|   This file is an IBIS representation of the   |
|   Integrated Device Technology Inc   |
|   IDT8T49N1012   |
|   FEMTOCLOCK NG 12-OUTPUT UNIVERSAL FREQUENCY SYNTHESIZER   |
[IBIS Ver]   4.1
[File name]   8t49n1012.ibs
[File Rev]   1.0
[Date]   16 Oct 2015
[Source]   Originated at Integrated Device Technology, Inc.
[Disclaimer]
IDT hereby grants the user of this IBIS model a non-exclusive,
nontransferable license to use this IBIS model under the following terms.
Before using this IBIS model, the user should read this license.
If the user does not accept these terms,  the IBIS model should be
returned to IDT within 30 days.
   The user is granted this license only to use the IBIS model and
is not granted rights to sell, load, rent, lease or license the IBIS
model in whole or in part, or in modified form to anyone other than
user. User may modify the IBIS model to suit its specific
applications but rights to derivative works and such modifications
shall belong to IDT.
   This IBIS model is provided on an "AS IS" basis and IDT makes
absolutely no warranty with respect to the information contained
herein. IDT DISCLAIMS AND CUSTOMER WAIVES ALL WARRANTIES, EXPRESS
OR IMPLIED, INCLUDING WARRANTIES OF MERCHANTABILITY OR FITNESS FOR
A PARTICULAR PURPOSE. The entire risk as to quality and performance
is with the Customer. ACCORDINGLY, IN NO EVENT SHALL THE COMPANY BE
LIABLE FOR ANY DAMAGES, WHETHER IN CONTRACT OR TORT,INCLUDING ANY
LOST PROFITS OR OTHER INCIDENTAL, CONSEQUENTIAL, EXEMPLARY, OR
PUNITIVE DAMAGES ARISING OUT OF THE USE OR APPLICATION OF THE IBIS
model provided in this package. Further, IDT reserves the right to
make changes without notice to any product herein to improve
reliability, function, or design. IDT does not convey any license
under patent rights or any other intellectual property rights,
including those of third parties.
   IDT is not obligated to provide maintenance or support
for the licensed IBIS model.
[Copyright] Copyright 2015 by Integrated Device Technology, Inc.
[Component]   IDT8T49N1012NLGI
[Manufacturer] Integrated Device Technology, Inc.
[Package]
|LD QFN 72
|lead + wire
|   Typ   Min   Max
R_pkg   7.8601440E-02   3.3809435E-02   1.3219826E-01
L_pkg   2.3894137E-09   1.4510419E-09   3.7197948E-09
C_pkg   6.1248861E-13   5.1617034E-13   1.0239547E-12
[Pin] signal_name model_name   R_pin   L_pin   C_pin
1  REF_OUT   CAK_IOCMOS35OHM0   1.0433593E-01   2.9865323E-09   5.7909691E-13
2  VCCA   POWER   9.7880543E-02   2.8166436E-09   5.6666836E-13
3  OSCI   CAK_INESD01_X   5.1811148E-02   1.8446542E-09   7.0153751E-13
4  OSCO   NC   4.9278689E-02   1.7780066E-09   6.8203455E-13
5  LOCK   CAK_IOCMOS35OHM0   8.6539992E-02   2.5181904E-09   5.4483440E-13
6  VCCO10   POWER   8.4441065E-02   2.4629522E-09   5.4079334E-13
7  Q11   CAK_OCELL_MULTOU   8.4441065E-02   2.4629522E-09   5.4079334E-13
8  nQ11   CAK_OCELL_MULTOU   4.8919175E-02   1.7685452E-09   6.7926586E-13
9  Q10   CAK_OCELL_MULTOU   4.9434655E-02   1.7821112E-09   6.8323567E-13
10 nQ10   CAK_OCELL_MULTOU   5.0386309E-02   1.8071563E-09   6.9056455E-13
11 NC   NC   5.0423318E-02   1.8081302E-09   6.9084956E-13
12 RSVD   NC   5.1361755E-02   1.8328274E-09   6.9807665E-13
13 VCCO8   POWER   9.0616246E-02   2.6254666E-09   5.5268241E-13
14 Q9   CAK_OCELL_MULTOU   5.4338319E-02   1.9111627E-09   7.2099976E-13
15 nQ9   CAK_OCELL_MULTOU   5.7534293E-02   1.9952722E-09   7.4561258E-13
16 Q8   CAK_OCELL_MULTOU   1.0684196E-01   3.0524842E-09   5.8392176E-13
17 nQ8   CAK_OCELL_MULTOU   6.3794065E-02   2.1600128E-09   7.9382033E-13
18 SA0/nCS   CAK_INESD01_PD   6.8504756E-02   2.2839856E-09   8.3009828E-13
19 SA1/SDI   CAK_INESD01_PD   1.3219826E-01   3.7197948E-09   6.3274024E-13
20 VCCO   POWER   1.1609415E-01   3.2959774E-09   6.0173501E-13
21 SCLK   CAK_IOCMOS35OHM0   7.5182199E-02   2.4597182E-09   8.8152259E-13
22 SDATA/SDO   CAK_IOCMOS35OHM0   6.9112757E-02   2.2999866E-09   8.3478062E-13
23 VEE   GND   1.1068558E-01   3.1536382E-09   5.9132189E-13
24 VCC   POWER   1.0047644E-01   2.8849608E-09   5.7166624E-13
25 NC   NC   9.3143418E-02   2.6919750E-09   5.5754797E-13
26 NC   NC   8.5715225E-02   2.4964847E-09   5.4324648E-13
27 VCCO7   POWER   4.6492456E-02   1.7046804E-09   6.6057722E-13
28 Q7   CAK_OCELL_MULTOU   4.4242850E-02   1.6454767E-09   6.4325256E-13
29 nQ7   CAK_OCELL_MULTOU   7.3021210E-02   2.1624120E-09   5.1880670E-13
30 NC   NC   7.3058219E-02   2.1633860E-09   5.1887795E-13
31 OE0   CAK_INESD01_PD_5   7.3338428E-02   2.1707603E-09   5.1941744E-13
32 NC   NC   7.3808968E-02   2.1831437E-09   5.2032337E-13
33 Q6   CAK_OCELL_MULTOU   8.4351186E-02   2.4605869E-09   5.4062029E-13
34 nQ6   CAK_OCELL_MULTOU   9.5194762E-02   2.7459609E-09   5.6149742E-13
35 VCCO6   POWER   1.0813726E-01   3.0865732E-09   5.8641562E-13
36 OE1   CAK_INESD01_PD_5   6.5747601E-02   2.2114246E-09   8.0886489E-13
37 nQ3   CAK_OCELL_MULTOU   4.9113451E-02   1.8538029E-09   1.0239547E-12
38 Q3   CAK_OCELL_MULTOU   9.7737794E-02   2.8128868E-09   5.6639352E-13
39 VCCO3   POWER   9.2530129E-02   2.6758349E-09   5.5636721E-13
40 NC   NC   9.2128319E-02   2.6652603E-09   5.5559360E-13
41 nQ2   CAK_OCELL_MULTOU   9.3656254E-02   2.7054715E-09   5.5853533E-13
42 Q2   CAK_OCELL_MULTOU   8.7877595E-02   2.5533926E-09   5.4740969E-13
43 VCCO2   POWER   4.9646134E-02   1.7876768E-09   6.8486431E-13
44 NC   NC   8.2659356E-02   2.4160624E-09   5.3736301E-13
45 nI2C/SPI   CAK_INESD01_PD_5   8.3494697E-02   2.4380463E-09   5.3897130E-13
46 NC   NC   3.7649538E-02   1.5521032E-09   8.2531156E-13
47 nQ1   CAK_OCELL_MULTOU   8.4081551E-02   2.4534908E-09   5.4010117E-13
48 Q1   CAK_OCELL_MULTOU   8.3891220E-02   2.4484818E-09   5.3973472E-13
49 VCCO1   POWER   8.3351949E-02   2.4342896E-09   5.3869646E-13
50 VCCO0   POWER   8.5186528E-02   2.4825708E-09   5.4222858E-13
51 nQ0   CAK_OCELL_MULTOU   9.1160804E-02   2.6397979E-09   5.5373085E-13
52 Q0   CAK_OCELL_MULTOU   9.8874493E-02   2.8428017E-09   5.6858201E-13
53 NC   NC   1.0953831E-01   3.1234451E-09   5.8911305E-13
54 PLL_BYP   CAK_INESD01_PD_5   1.2195212E-01   3.4501434E-09   6.1301334E-13
55 nQ5   CAK_OCELL_MULTOU   1.2167719E-01   3.4429082E-09   6.1248403E-13
56 Q5   CAK_OCELL_MULTOU   8.8147231E-02   2.5604887E-09   5.4792882E-13
57 VCCO5   POWER   7.9159382E-02   2.3239524E-09   5.3062452E-13
58 nRST   CAK_INESD01_PU_5   7.4469839E-02   2.2005361E-09   5.2159574E-13
59 nQ4   CAK_OCELL_MULTOU   7.7462265E-02   2.2792887E-09   5.2735706E-13
60 Q4   CAK_OCELL_MULTOU   4.4171476E-02   1.6435984E-09   6.4270289E-13
61 VCCO4   POWER   3.3809435E-02   1.4510419E-09   7.5877144E-13
62 LOS   CAK_IOCMOS35OHM0   7.5040832E-02   2.2155631E-09   5.2269508E-13
63 VCCA   POWER   7.4718327E-02   2.2070756E-09   5.2207416E-13
64 CAP_REF   NC   7.1651884E-02   2.1263750E-09   5.1617034E-13
65 CAP   NC   4.4782121E-02   1.6596689E-09   6.4740559E-13
66 VCCA   POWER   4.5897672E-02   1.6890272E-09   6.5599667E-13
67 VCCA_PDCP0   POWER   8.0169193E-02   2.3505279E-09   5.3256871E-13
68 VCCA   POWER   7.4554431E-02   2.2027623E-09   5.2175861E-13
69 VCCCS   POWER   8.1015108E-02   2.3727901E-09   5.3419735E-13
70 CLK_SEL   CAK_INESD01_PU_5   8.9516556E-02   2.5965257E-09   5.5056518E-13
71 nCLK   CAK_INESD02_PMID   9.8779328E-02   2.8402972E-09   5.6839879E-13
72 CLK   CAK_INESD02_PD   1.0886687E-01   3.1057744E-09   5.8782032E-13
[Diff Pin]   inv_pin vdiff   tdelay_typ   tdelay_min   tdelay_max
| Inputs
72   71   0.15   NA   NA   NA
|Outputs
7   8   NA   0   0   0
9   10   NA   0   0   0
14   15   NA   0   0   0
16   17   NA   0   0   0
28   29   NA   0   0   0
33   34   NA   0   0   0
38   37   NA   0   0   0
42   41   NA   0   0   0
48   47   NA   0   0   0
52   51   NA   0   0   0
56   55   NA   0   0   0
60   59   NA   0   0   0
[Model Selector] CAK_INESD01
CAK_INESD01_2v5   Buffer selection for 2v5
CAK_INESD01_3v3   Buffer selection for 3v3
[Model Selector] CAK_INESD01_X
CAK_INESD01X_2v5   Buffer selection for 2v5
CAK_INESD01X_3v3   Buffer selection for 3v3
[Model Selector] CAK_INESD02_PD
CAK_INESD02_PD_2v5  Buffer selection for 2v5
CAK_INESD02_PD_3v3  Buffer selection for 3v3
[Model Selector] CAK_INESD02_PMID
CAK_INESD02_PMID_2v5  Buffer selection for 2v5
CAK_INESD02_PMID_3v3  Buffer selection for 3v3
[Model Selector] CAK_IOCMOS35OHM0
CAK_IOCMOS35OHM0_2v5  Buffer selection for 2v5
CAK_IOCMOS35OHM0_3v3  Buffer selection for 3v3
[Model Selector] CAK_IOCMOS25OHM0
CAK_IOCMOS25OHM0_2v5  Buffer selection for 2v5
CAK_IOCMOS25OHM0_3v3  Buffer selection for 3v3
[Model Selector] CAK_OCELL_MULTOU
CAK_OCELL_LVPECL_2v5  Buffer selection for LVPECL 2.5V
CAK_OCELL_LVPECL_3v3  Buffer selection for LVPECL 3.3V
CAK_OCELL_LVDS_2v5   Buffer selection for LVDS 2.5V
CAK_OCELL_LVDS_3v3   Buffer selection for LVDS 3.3V
CAK_OCELL_CMOS_1v8   Buffer selection for CMOS 1.8V
CAK_OCELL_CMOS_2v5   Buffer selection for CMOS 2.5V
CAK_OCELL_CMOS_3v3   Buffer selection for CMOS 3.3V
CAK_OCELL_HCSL_2v5   Buffer selection for HCSL 2.5V
CAK_OCELL_HCSL_3v3   Buffer selection for HCSL 3.3V
[Model Selector] CAK_INESD01_PU_5
CAK_INESD01_PU_5_2v5  Buffer selection for 2v5
CAK_INESD01_PU_5_3v3  Buffer selection for 3v3
[Model Selector] OUTPUT_OD01
OUTPUT_OD01_2v5  Buffer selection for 2v5
OUTPUT_OD01_3v3  Buffer selection for 3v3
[Model Selector] CAK_INESD01_PD_5
CAK_INESD01_PD_5_2v5  Buffer selection for 2v5
CAK_INESD01_PD_5_3v3  Buffer selection for 3v3
[Model Selector] CAK_INESD01_PD
CAK_INESD01_PD_2v5  Buffer selection for 2v5
CAK_INESD01_PD_3v3  Buffer selection for 3v3
| Models and submodels in the file (29): CAK_INESD01_3v3 (Input), CAK_INESD01X_3v3 (Input), CAK_INESD01_2v5 (Input), CAK_INESD01X_2v5 (Input), CAK_OCELL_CMOS_1v8 (Output), CAK_INESD02_PD_2v5 (Input), CAK_INESD02_PMID_2v5 (Input), CAK_IOCMOS35OHM0_2v5 (I/O), CAK_IOCMOS25OHM0_2v5 (I/O), CAK_OCELL_LVPECL_2v5 (Output_ECL), CAK_OCELL_CMOS_2v5 (Output), CAK_OCELL_LVDS_2v5 (Output), CAK_INESD01_PU_5_2v5 (Input), OUTPUT_OD01_2v5 (Open_drain), CAK_INESD01_PD_5_2v5 (Input), CAK_INESD02_PD_3v3 (Input), CAK_INESD02_PMID_3v3 (Input), CAK_IOCMOS35OHM0_3v3 (Output), CAK_IOCMOS25OHM0_3v3 (I/O), CAK_OCELL_LVPECL_3v3 (Output_ECL), CAK_OCELL_CMOS_3v3 (Output), CAK_OCELL_LVDS_3v3 (Output), CAK_INESD01_PU_5_3v3 (Input), OUTPUT_OD01_3v3 (Open_drain), CAK_INESD01_PD_5_3v3 (Input), CAK_OCELL_HCSL_3v3 (Open_source), CAK_OCELL_HCSL_2v5 (Open_source), CAK_INESD01_PD_3v3 (Input), CAK_INESD01_PD_2v5 (Input)
